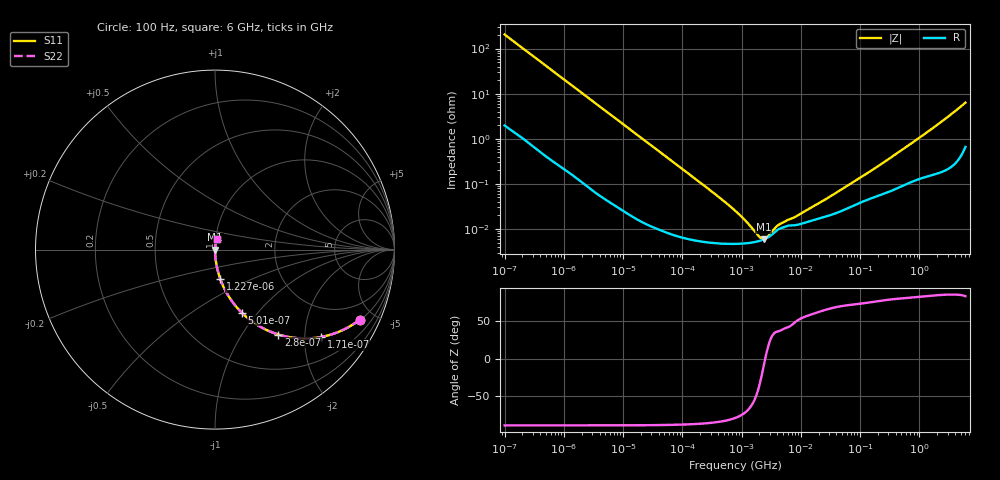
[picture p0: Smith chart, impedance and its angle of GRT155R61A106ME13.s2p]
!Murata Part Number: GRT155R61A106ME13
!These Parameters are Measured in Series Mode Connection
!Data Generated on Jun 19, 2026
!  o--ll--o
!Port1  Port2
!  o------o
!Operation Temp=25[degC], DC Bias Voltage=0[V]
!Freq. Start=100[Hz] Stop=6[GHz] 401[Steps]
# Hz S RI R 50
!Freq.(Hz) S11(Real) S11(Imag) S21(Real) S21(Imag) S12(Real) S12(Imag) S22(Real) S22(Imag)
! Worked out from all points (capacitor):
!   401 points, 100 Hz to 6 GHz, reference 50 ohm
!   read as one part in series: C = 7.74 uF near 109 Hz
!   lowest |Z| = 5.95 mohm at 2.373 MHz (marker M1)
!   series resonance near 2.505 MHz, so ESL is about 520 pH
!   S11 on the Smith chart (normalised r, x): 100 Hz: 1.04, -4.10; 171 Hz: 1.02, -2.41; 280 Hz: 1.01, -1.48; 501 Hz: 1.01, -0.83; 1.227 kHz: 1.00, -0.34; 6 GHz: 1.01, +0.13
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100  0.8057 -0.3909  0.1943 0.3909  0.1943 0.3909  0.8057 -0.3909
171  0.5905 -0.4868  0.4095 0.4868  0.4095 0.4868  0.5905 -0.4868
280  0.3537 -0.4732  0.6463 0.4732  0.6463 0.4732  0.3537 -0.4732
501  0.1485 -0.3507  0.8515 0.3507  0.8515 0.3507  0.1485 -0.3507
750  0.0735 -0.2559  0.9265 0.2559  0.9265 0.2559  0.0735 -0.2559
1227  0.0297 -0.1645  0.9703 0.1645  0.9703 0.1645  0.0297 -0.1645
2008  0.0118 -0.1028  0.9882 0.1028  0.9882 0.1028  0.0118 -0.1028
6433  0.00143 -0.0327  0.9986 0.0327  0.9986 0.0327  0.00143 -0.0327
40335  0.000124 -0.00528  0.9999 0.00528  0.9999 0.00528  0.000124 -0.00528
316350  4.96e-05 -0.000671  1 0.000671  1 0.000671  4.96e-05 -0.000671
774597  4.68e-05 -0.000252  1 0.000252  1 0.000252  4.68e-05 -0.000252
1516199  5.02e-05 -9.01e-05  0.9999 9.01e-05  0.9999 9.01e-05  5.02e-05 -9.01e-05
1734173  5.19e-05 -6.47e-05  0.9999 6.47e-05  0.9999 6.47e-05  5.19e-05 -6.47e-05
2372521  5.88e-05 -9.2e-06  0.9999 9.2e-06  0.9999 9.2e-06  5.88e-05 -9.2e-06
3549919  8.28e-05 5.63e-05  0.9999 -5.63e-05  0.9999 -5.63e-05  8.28e-05 5.63e-05
4643984  0.000105 8.22e-05  0.9999 -8.22e-05  0.9999 -8.22e-05  0.000105 8.22e-05
7947587  0.000121 0.000139  0.9999 -0.000139  0.9999 -0.000139  0.000121 0.000139
1.555665e7  0.000154 0.000266  0.9998 -0.000266  0.9998 -0.000266  0.000154 0.000266
3.80911e7  0.000221 0.000576  0.9998 -0.000576  0.9998 -0.000576  0.000221 0.000576
3.124326e8  0.000685 0.00358  0.9993 -0.00358  0.9993 -0.00358  0.000685 0.00358
1.497423e9  0.00174 0.0152  0.9983 -0.0152  0.9983 -0.0152  0.00174 0.0152
6e9  0.0104 0.0617  0.9896 -0.0617  0.9896 -0.0617  0.0104 0.0617
